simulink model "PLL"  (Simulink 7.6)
settings: Solver=FixedStepDiscrete  StartTime=0.0  StopTime=0.02  FixedStep=Ts  RelTol=1e-3
InitFcn:
  | f=60;
  | Ts=2e-5;
libraries: powerlib_extras x1

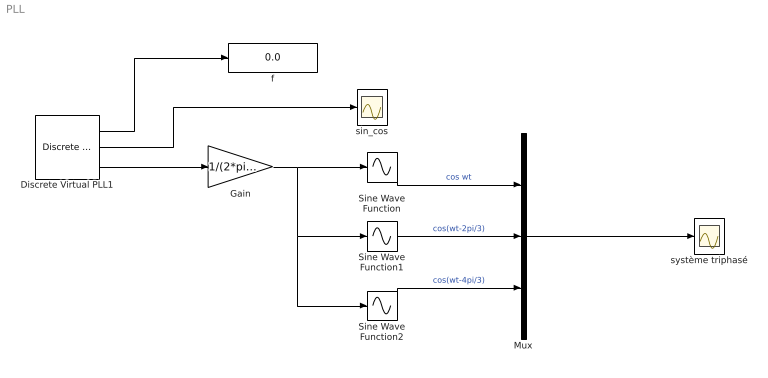
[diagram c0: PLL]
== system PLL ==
  Discrete Virtual PLL1 : powerlib_extras/Discrete  Control Blocks/Discrete Virtual PLL  DialogController=POWERSYS.PowerSysDialog  SystemSampleTime=-1  Freq=f  Phase=0  Ts=Ts
  Gain : Gain  Gain=1/(2*pi*f)
  Mux : Mux  Inputs=3
  Sine Wave Function : Sin  TimeSource=Use external signal  Frequency=2*pi*f  SampleTime=0
  Sine Wave Function1 : Sin  TimeSource=Use external signal  Frequency=2*pi*f  Phase=-2*pi/3  SampleTime=0
  Sine Wave Function2 : Sin  TimeSource=Use external signal  Frequency=2*pi*f  Phase=-4*pi/3  SampleTime=0
  f : Display
  sin_cos : Scope
  système triphasé : Scope
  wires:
  Discrete Virtual PLL1/3 -> Gain/1
  Gain/1 -> Sine Wave Function/1, Sine Wave Function1/1, Sine Wave Function2/1
  Sine Wave Function1/1 -> Mux/2  "cos(wt-2pi/3)"
  Sine Wave Function/1 -> Mux/1  "cos wt"
  Sine Wave Function2/1 -> Mux/3  "cos(wt-4pi/3)"
  Mux/1 -> système triphasé/1
  Discrete Virtual PLL1/2 -> sin_cos/1
  Discrete Virtual PLL1/1 -> f/1
